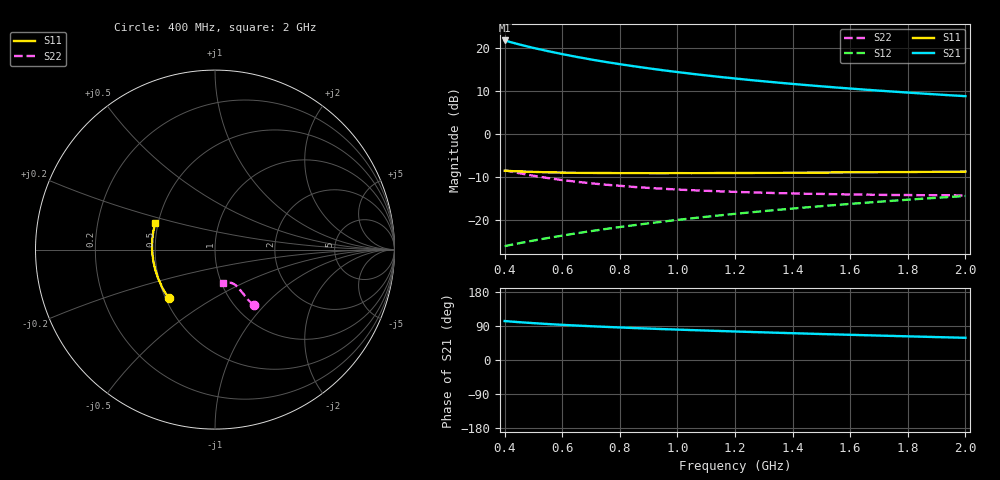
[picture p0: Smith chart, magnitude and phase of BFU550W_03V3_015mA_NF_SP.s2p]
! Filename:  P:\Prog\Test\Noise\ATS_data\Testdata_Net\06 Compressed Noise after Statistics\BFU550W_APM2013_11_D05_03p3V_015mA_NF_CM01_D.sf
! Date/Time: Tue 26/Mar/2013 16:25:23
! BFU550W_APM2013_11_D05_03p3V_1to35mA_NF_CM01_Bias7_R.sf
! Noise Parameter Data File
! BFU550W_APM2013_11_D05_03p3V_1to35mA_NF_CM01
! Date/time: Mon Mar 25 12:16:07 2013
! VAR V_out= 3.300000
! VAR I_out= 15.000000
! VAR V_in= 0.835500
! VAR I_in= 0.161000
! Device data file deembeded for feedlines and parallel
! Original file: \06 Compressed Noise after Statistics\BFU550W_APM2013_11_D05_03p3V_015mA_NF_CM01_R.sf
! Feed-files: PR019V01_070313_Feed1.s2p, PR019V01_070313_Feed2.s2p
! Parallel-file: PR019V01_070313_Par.s2p
# MHz S MA R 50
!  Freq-MHz  S11-mag  S11-arg  S21-mag  S21-arg  S12-mag  S12-arg  S22-mag  S22-arg
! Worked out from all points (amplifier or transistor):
!   37 points, 400 MHz to 2 GHz, reference 50 ohm
!   highest |S21| = 21.6 dB at 400 MHz (marker M1)
!   |S21| within 3 dB of that: start of sweep to 588.4 MHz
!   unconditionally stable (mu >= 1): 1.143 GHz to end of sweep
!   at 500 MHz: K = 0.85, MSG = 22.3 dB, |S12| = -24.8 dB
!   at 1.1 GHz: K = 1.00, MSG = 16.4 dB, |S12| = -19.3 dB
!   at 2 GHz: K = 1.01, MAG = 10.9 dB, |S12| = -14.4 dB
!   lowest NFmin = 0.79 dB at 420 MHz
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400  0.3725 -133.5  12.09 102.8  0.0497 62.3  0.3779 -55.3
420  0.37 -136.2  11.59 101.6  0.05136 62.5  0.3661 -55.7
433  0.3676 -137.7  11.28 100.8  0.05237 62.7  0.3585 -55.9
460  0.3655 -140.6  10.68 99.3  0.05453 63.1  0.3443 -56.3
500  0.3619 -144.9  9.91 97.3  0.05773 63.6  0.326 -56.8
550  0.3565 -149.2  9.104 94.9  0.06183 64.3  0.3067 -57.1
600  0.3552 -153.3  8.402 92.8  0.06591 64.8  0.2903 -57.4
650  0.3523 -156.8  7.798 90.9  0.0701 65.4  0.2778 -57.8
700  0.3515 -160.1  7.277 89.1  0.07432 65.8  0.2665 -58.1
750  0.351 -162.9  6.821 87.5  0.07857 66.1  0.2568 -58.4
800  0.3493 -165.8  6.419 85.9  0.08285 66.4  0.2492 -58.9
850  0.3497 -168.4  6.063 84.3  0.08709 66.7  0.2416 -59.1
950  0.3485 -172.8  5.457 81.5  0.09583 67.0  0.2304 -59.9
1050  0.3491 -176.9  4.965 78.9  0.1046 67.2  0.2217 -60.8
1150  0.3508 179.2  4.555 76.5  0.1134 67.2  0.2149 -61.9
1200  0.3502 177.7  4.38 75.3  0.1179 67.2  0.2122 -62.6
1250  0.3511 175.8  4.212 74.1  0.1223 67.1  0.2093 -63.0
1350  0.3523 172.9  3.92 71.8  0.1313 66.9  0.2049 -64.4
1500  0.3546 168.5  3.553 68.5  0.1447 66.3  0.2006 -66.8
1650  0.3574 164.3  3.253 65.5  0.1583 65.7  0.197 -69.2
1750  0.3594 162.0  3.083 63.4  0.1673 65.2  0.1949 -71.1
2000  0.3647 156.0  2.731 58.6  0.1899 63.8  0.193 -76.3
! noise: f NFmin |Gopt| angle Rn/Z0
400  0.8308  0.2384  -177.7  0.0624
460  0.8325  0.2411  -177.2  0.0627
600  0.8579  0.2431  -169  0.0671
800  0.8973  0.2683  -170.9  0.061
1000  0.9232  0.2756  -169.9  0.0616
1200  0.9418  0.2893  -165.3  0.0639
1400  0.9848  0.3065  -163.4  0.0651
1600  1.009  0.3158  -159.4  0.0683
1800  1.038  0.3297  -155.7  0.0714
2000  1.075  0.3426  -153  0.0751
